| TEXAS INSTRUMENTS INCORPORATED
| Standard Linear and Logic Group
| IBIS Model of SN74LV244AT
| Octal Buffer/Driver With 3-State Outputs
| This file contains package information for the following:
|  SOIC 20-pin (DW) package as [Component] LV244AT_DW
|  TVSOP 20-pin (DGV) package as [Component] LV244AT_DGV
|  TSSOP 20-pin (PW) package as [Component] LV244AT_PW
|  SSOP 20-pin (DB) package as [Component] LV244AT_DB
|  QFN 20-pin (RGY) package as [Component] LV244AT_RGY
|  SOP 20-pin (NS) package as [Component] LV244AT_NS
| This device can be powered at the following Vccs:
|  5 volt Vcc
| This file provides unique models under the [Model Selector] for each Vcc.
| For operation at a specific Vcc, select the appropriate model after each
| [Model Selector] keyword.
[IBIS Ver]   3.2
[Comment char]  |_char
[File Name]   sn74lv244at.ibs
[File Rev]   2.1 | x_die
[Date]   June 15, 2004
[Source]   Data created from TI-SPICE simulations at TI-SLL.
[Notes]   The following is an IBIS list for the LV244AT.
   Please contact sllibis@ti.com with questions and
   comments concerning SLL IBIS models.
   - FILE REV HISTORY
   - 2.1 Release IBIS file on 06/17/04
   - Non-monotonice data in pullup due to Ioff circuitry at output.
   - Power clamp data deleted as there is no power-clamp diode.
[Disclaimer] Property of Texas Instruments Incorporated.  Unauthorized
   reproduction and/or distribution is strictly prohibited.
   This product is protected under copyright law.
   Created  2003, (C) Copyright  2003, Texas Instruments
   Incorporated, All Rights Reserved
   UNLESS THERE IS A SIGNED, WRITTEN AGREEMENT TO THE
   CONTRARY, TEXAS INSTRUMENTS (TI) IS PROVIDING THE IBIS
   MODELS  AND WITHOUT ANY WARRANTY, EXPRESSED OR
   IMPLIED.  TI assumes no liability for:
   1) the accuracy of the IBIS models provided to your
   company;
   2) the proper functioning of these IBIS Models in your
   design or for any resulting applications; or
   3) infringement of patents, copyrights or intellectual
   property rights resulting from your use of these IBIS
   models.
   TI provides IBIS Models as a service to our customers.
   You and your company shall not distribute, sell or give
   these models to anyone else without prior written
   permission from TI.
   TI reserves the right to make changes to our products or
   to discontinue any semiconductor product or service
   without notice, and advises our customers to obtain the
   latest version of relevant information to verify, before
   placing orders, that the information being relied on is
   current.
   Please be aware that your receipt and use of the IBIS
   information provided shall serve as acceptance of these
   terms and conditions.  If you do not accept these terms,
   you should return or destroy the IBIS models and any
   other accompanying information immediately.
| Component LV244AT_DGV 20-pin TVSOP
[Component]   LV244AT_DGV
[Manufacturer]   Texas Instruments, Inc.
[Package]
|   typ   min   max
R_pkg   4.400e-02   3.800e-02   4.800e-02
L_pkg   2.561e-09   2.236e-09   2.961e-09
C_pkg   3.420e-13   2.640e-13   4.460e-13
[Pin]   signal_name   model_name   R_pin   L_pin   C_pin
1   1NOE   LV244AT_IN   4.400e-02   2.935e-09   4.170e-13
2   1A1   LV244AT_IN   4.200e-02   2.869e-09   4.460e-13
3   2Y4   LV244AT_OUT   4.300e-02   2.399e-09   3.160e-13
4   1A2   LV244AT_IN   4.400e-02   2.236e-09   2.650e-13
5   2Y3   LV244AT_OUT   4.600e-02   2.278e-09   2.640e-13
6   1A3   LV244AT_IN   4.500e-02   2.274e-09   2.640e-13
7   2Y2   LV244AT_OUT   4.400e-02   2.285e-09   2.690e-13
8   1A4   LV244AT_IN   4.300e-02   2.452e-09   3.200e-13
9   2Y1   LV244AT_OUT   4.400e-02   2.900e-09   4.460e-13
10   GND   GND   4.400e-02   2.961e-09   4.180e-13
11   2A1   LV244AT_IN   4.500e-02   2.954e-09   4.180e-13
12   1Y4   LV244AT_OUT   4.200e-02   2.847e-09   4.430e-13
13   2A2   LV244AT_IN   4.500e-02   2.453e-09   3.190e-13
14   1Y3   LV244AT_OUT   4.500e-02   2.297e-09   2.690e-13
15   2A3   LV244AT_IN   4.800e-02   2.334e-09   2.680e-13
16   1Y2   LV244AT_OUT   4.800e-02   2.335e-09   2.670e-13
17   2A4   LV244AT_IN   4.600e-02   2.299e-09   2.680e-13
18   1Y1   LV244AT_OUT   4.600e-02   2.457e-09   3.200e-13
19   2NOE   LV244AT_IN   4.300e-02   2.848e-09   4.410e-13
20   VCC   POWER   3.800e-02   2.812e-09   4.080e-13
| Component LV244AT_PW 20-pin TSSOP
[Component]   LV244AT_PW
[Manufacturer]   Texas Instruments, Inc.
[Package]
|   typ   min   max
R_pkg   4.500e-02   3.600e-02   5.700e-02
L_pkg   2.694e-09   2.290e-09   3.177e-09
C_pkg   1.560e-13   7.600e-14   2.590e-13
[Pin]   signal_name   model_name   R_pin   L_pin   C_pin
1   1NOE   LV244AT_IN   3.600e-02   3.045e-09   2.590e-13
2   1A1   LV244AT_IN   5.100e-02   3.013e-09   1.890e-13
3   2Y4   LV244AT_OUT   4.400e-02   2.695e-09   1.640e-13
4   1A2   LV244AT_IN   4.700e-02   2.362e-09   7.900e-14
5   2Y3   LV244AT_OUT   4.700e-02   2.333e-09   8.600e-14
6   1A3   LV244AT_IN   4.700e-02   2.298e-09   8.500e-14
7   2Y2   LV244AT_OUT   4.700e-02   2.351e-09   7.900e-14
8   1A4   LV244AT_IN   4.400e-02   2.706e-09   1.650e-13
9   2Y1   LV244AT_OUT   4.900e-02   2.999e-09   1.880e-13
10   GND   GND   3.900e-02   3.039e-09   2.570e-13
11   2A1   LV244AT_IN   3.800e-02   3.044e-09   2.580e-13
12   1Y4   LV244AT_OUT   5.700e-02   3.177e-09   1.990e-13
13   2A2   LV244AT_IN   4.400e-02   2.825e-09   1.730e-13
14   1Y3   LV244AT_OUT   4.700e-02   2.429e-09   8.300e-14
15   2A3   LV244AT_IN   4.900e-02   2.383e-09   9.000e-14
16   1Y2   LV244AT_OUT   4.900e-02   2.347e-09   8.900e-14
17   2A4   LV244AT_IN   4.700e-02   2.290e-09   7.600e-14
18   1Y1   LV244AT_OUT   4.500e-02   2.613e-09   1.580e-13
19   2NOE   LV244AT_IN   4.400e-02   2.883e-09   1.810e-13
20   VCC   POWER   3.900e-02   3.044e-09   2.560e-13
| Component LV244AT_DW 20-pin SOIC
[Component]   LV244AT_DW
[Manufacturer]   Texas Instruments, Inc.
[Package]
|   typ   min   max
R_pkg   3.800e-02   3.300e-02   4.500e-02
L_pkg   5.012e-09   4.110e-09   6.349e-09
C_pkg   7.170e-13   5.300e-13   8.680e-13
[Pin]   signal_name   model_name   R_pin   L_pin   C_pin
1   NOE1   LV244AT_IN   4.200e-02   6.336e-09   8.650e-13
2   1A1   LV244AT_IN   4.300e-02   5.542e-09   8.670e-13
3   2Y4   LV244AT_OUT   3.400e-02   4.714e-09   7.320e-13
4   1A2   LV244AT_IN   3.400e-02   4.377e-09   5.910e-13
5   2Y3   LV244AT_OUT   3.600e-02   4.130e-09   5.330e-13
6   1A3   LV244AT_IN   3.500e-02   4.111e-09   5.300e-13
7   2Y2   LV244AT_OUT   3.400e-02   4.284e-09   5.830e-13
8   1A4   LV244AT_IN   3.400e-02   4.634e-09   7.260e-13
9   2Y1   LV244AT_OUT   4.000e-02   5.518e-09   8.650e-13
10   GND   GND   4.300e-02   6.349e-09   8.660e-13
11   2A1   LV244AT_IN   4.100e-02   6.281e-09   8.610e-13
12   1Y4   LV244AT_OUT   4.500e-02   5.561e-09   8.680e-13
13   2A2   LV244AT_IN   3.300e-02   4.778e-09   7.420e-13
14   1Y3   LV244AT_OUT   3.500e-02   4.414e-09   5.960e-13
15   2A3   LV244AT_IN   3.500e-02   4.110e-09   5.330e-13
16   1Y2   LV244AT_OUT   3.600e-02   4.130e-09   5.330e-13
17   2A4   LV244AT_IN   3.400e-02   4.377e-09   5.910e-13
18   1Y1   LV244AT_OUT   3.400e-02   4.714e-09   7.310e-13
19   NOE2   LV244AT_IN   4.300e-02   5.569e-09   8.680e-13
20   VCC   POWER   4.200e-02   6.308e-09   8.640e-13
| Component LV244AT_DB 20-pin SSOP
[Component]   LV244AT_DB
[Manufacturer]   Texas Instruments, Inc.
[Package]
|   typ   min   max
R_pkg   4.000e-02   3.500e-02   5.100e-02
L_pkg   3.495e-09   3.035e-09   4.314e-09
C_pkg   4.200e-13   3.460e-13   5.020e-13
[Pin]   signal_name   model_name   R_pin   L_pin   C_pin
1   NOE1   LV244AT_IN   4.900e-02   4.310e-09   5.020e-13
2   1A1   LV244AT_IN   4.800e-02   3.903e-09   4.870e-13
3   2Y4   LV244AT_OUT   3.500e-02   3.189e-09   3.960e-13
4   1A2   LV244AT_IN   3.500e-02   3.036e-09   3.470e-13
5   2Y3   LV244AT_OUT   3.500e-02   3.035e-09   3.670e-13
6   1A3   LV244AT_IN   3.500e-02   3.035e-09   3.670e-13
7   2Y2   LV244AT_OUT   3.500e-02   3.036e-09   3.470e-13
8   1A4   LV244AT_IN   3.500e-02   3.189e-09   3.970e-13
9   2Y1   LV244AT_OUT   4.700e-02   3.899e-09   4.880e-13
10   GND   GND   5.100e-02   4.314e-09   5.000e-13
11   2A1   LV244AT_IN   5.100e-02   4.314e-09   5.000e-13
12   1Y4   LV244AT_OUT   4.700e-02   3.899e-09   4.880e-13
13   2A2   LV244AT_IN   3.500e-02   3.189e-09   3.970e-13
14   1Y3   LV244AT_OUT   3.500e-02   3.036e-09   3.460e-13
15   2A3   LV244AT_IN   3.500e-02   3.035e-09   3.670e-13
16   1Y2   LV244AT_OUT   3.500e-02   3.035e-09   3.670e-13
17   2A4   LV244AT_IN   3.500e-02   3.036e-09   3.460e-13
18   1Y1   LV244AT_OUT   3.500e-02   3.189e-09   3.970e-13
19   NOE2   LV244AT_IN   4.700e-02   3.899e-09   4.880e-13
20   VCC   POWER   5.100e-02   4.314e-09   5.020e-13
| Component LV244AT_RGY 20-pin QFN
[Component]   LV244AT_RGY
[Manufacturer]   Texas Instruments, Inc.
[Package]
|   typ   min   max
R_pkg   0.046   0.035   0.058
L_pkg   1.131nH   0.880nH   1.396nH
C_pkg   0.165pF   0.142pF   0.175pF
[Pin]   signal_name   model_name   R_pin   L_pin   C_pin
1   NOE1   LV244AT_IN   0.053   1.289nH   0.142pF
2   1A1   LV244AT_IN   0.058   1.386nH   0.172pF
3   2Y4   LV244AT_OUT   0.046   1.111nH   0.173pF
4   1A2   LV244AT_IN   0.039   0.965nH   0.161pF
5   2Y3   LV244AT_OUT   0.035   0.881nH   0.165pF
6   1A3   LV244AT_IN   0.035   0.880nH   0.165pF
7   2Y2   LV244AT_OUT   0.039   0.961nH   0.161pF
8   1A4   LV244AT_IN   0.045   1.105nH   0.172pF
9   2Y1   LV244AT_OUT   0.058   1.386nH   0.172pF
10   GND   GND   0.056   1.352nH   0.159pF
11   2A1   LV244AT_IN   0.053   1.287nH   0.155pF
12   1Y4   LV244AT_OUT   0.058   1.396nH   0.172pF
13   2A2   LV244AT_IN   0.047   1.129nH   0.175pF
14   1Y3   LV244AT_OUT   0.040   0.976nH   0.164pF
15   2A3   LV244AT_IN   0.035   0.884nH   0.169pF
16   1Y2   LV244AT_OUT   0.035   0.881nH   0.168pF
17   2A4   LV244AT_IN   0.039   0.967nH   0.162pF
18   1Y1   LV244AT_OUT   0.046   1.118nH   0.174pF
19   NOE2   LV244AT_IN   0.058   1.396nH   0.175pF
20   VCC   POWER   0.052   1.276nH   0.144pF
| Component LV244AT_NS 20-pin SOP
[Component]   LV244AT_NS
[Manufacturer]   Texas Instruments, Inc.
[Package]
|   typ   min   max
R_pkg   4.400e-02   2.900e-02   5.800e-02
L_pkg   3.666e-09   2.317e-09   5.115e-09
C_pkg   5.480e-13   3.160e-13   7.250e-13
[Pin]   signal_name   model_name   R_pin   L_pin   C_pin
1   NOE1   LV244AT_IN   5.800e-02   5.115e-09   7.250e-13
2   1A1   LV244AT_IN   5.300e-02   4.591e-09   7.240e-13
3   2Y4   LV244AT_OUT   4.900e-02   3.754e-09   5.720e-13
4   1A2   LV244AT_IN   2.900e-02   2.549e-09   3.880e-13
5   2Y3   LV244AT_OUT   3.100e-02   2.317e-09   3.160e-13
6   1A3   LV244AT_IN   3.100e-02   2.317e-09   3.160e-13
7   2Y2   LV244AT_OUT   2.900e-02   2.556e-09   3.990e-13
8   1A4   LV244AT_IN   4.900e-02   3.754e-09   5.790e-13
9   2Y1   LV244AT_OUT   5.300e-02   4.591e-09   7.240e-13
10   GND   GND   5.800e-02   5.115e-09   7.250e-13
11   2A1   LV244AT_IN   5.800e-02   5.115e-09   7.250e-13
12   1Y4   LV244AT_OUT   5.300e-02   4.591e-09   7.240e-13
13   2A2   LV244AT_IN   4.900e-02   3.754e-09   5.790e-13
14   1Y3   LV244AT_OUT   2.900e-02   2.557e-09   3.990e-13
15   2A3   LV244AT_IN   3.100e-02   2.317e-09   3.160e-13
16   1Y2   LV244AT_OUT   3.100e-02   2.317e-09   3.160e-13
17   2A4   LV244AT_IN   2.900e-02   2.557e-09   3.990e-13
18   1Y1   LV244AT_OUT   4.900e-02   3.754e-09   5.790e-13
19   NOE2   LV244AT_IN   5.300e-02   4.591e-09   7.240e-13
20   VCC   POWER   5.800e-02   5.115e-09   7.250e-13
| Models and submodels in the file (2): LV244AT_IN (Input), LV244AT_OUT (3-state)
